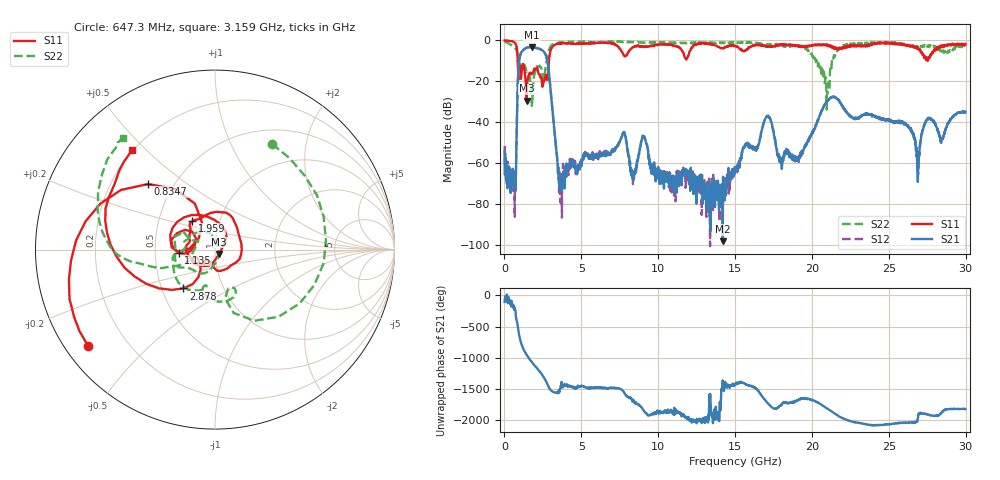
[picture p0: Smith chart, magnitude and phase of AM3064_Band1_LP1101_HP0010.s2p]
# Hz S DB R 50.0
!freq dBS11 angS11 dBS21 angS21 dBS12 angS12 dBS22 angS22
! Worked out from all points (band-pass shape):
!   1600 points, 10 MHz to 29.98 GHz, reference 50 ohm
!   highest |S21| = -3.29 dB at 1.791 GHz (marker M1); lowest = -98.2 dB at 14.2 GHz (marker M2)
!   |S21| within 3 dB of the highest: 1.065 GHz to 2.629 GHz (1.565 GHz wide, 84.7 % of centre)
!   lowest |S11| = -29.5 dB at 1.435 GHz (marker M3), VSWR 1.07, Z = 52.2 - j2.6 ohm
!   |S11| at or under -10 dB: 865.9 MHz to 2.892 GHz (2.026 GHz wide, 108 % of centre)
!   |S22| runs from -33.8 to -0.4 dB; largest |S21 - S12| = 0.01
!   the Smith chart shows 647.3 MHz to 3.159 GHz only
!   S11 on the Smith chart (normalised r, x): 647.3 MHz: 0.07, -0.33; 834.7 MHz: 0.36, +0.36; 1.135 GHz: 0.66, -0.02; 1.959 GHz: 0.74, +0.25; 2.878 GHz: 0.65, -0.30; 3.159 GHz: 0.20, +0.45
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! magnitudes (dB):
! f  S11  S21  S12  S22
! 10 MHz  0.0  -54.2  -51.6  -0.4
! 647.3 MHz  -1.0  -64.1  -67.9  -3.5
! 834.7 MHz  -5.6  -30.5  -30.3  -6.9
! 1.135 GHz  -13.8  -5.4  -5.3  -12.8
! 1.435 GHz  -29.5  -3.6  -3.6  -15.5
! 1.791 GHz  -16.3  -3.3  -3.3  -32.6
! 1.959 GHz  -13.8  -3.5  -3.5  -16.2
! 2.878 GHz  -11.1  -14.7  -14.6  -5.1
! 3.159 GHz  -2.8  -37.0  -37.2  -1.9
! 3.628 GHz  -1.3  -70.8  -79.4  -1.2
! 5.015 GHz  -1.5  -61.3  -60.0  -0.7
! 7.732 GHz  -6.9  -45.2  -45.2  -0.6
! 10 GHz  -2.1  -61.9  -64.0  -1.0
! 14.2 GHz  -3.9  -98.2  -73.9  -1.2
! 15 GHz  -2.8  -64.4  -64.9  -1.3
! 17.09 GHz  -2.7  -37.1  -37.3  -2.0
! 17.99 GHz  -2.3  -57.7  -58.4  -2.4
! 19.99 GHz  -2.7  -45.7  -45.3  -7.0
! 20.98 GHz  -2.2  -29.8  -29.7  -26.3
! 25 GHz  -1.1  -39.0  -39.2  -1.2
! 26.89 GHz  -3.8  -69.2  -63.7  -3.3
! 29.98 GHz  -1.8  -35.0  -34.8  -2.8
